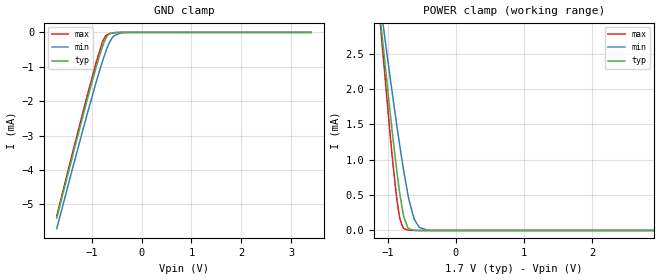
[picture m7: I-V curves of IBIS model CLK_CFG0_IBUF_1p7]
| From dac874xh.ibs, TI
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|   CLK_CFG0_IBUF_1p7 Model
[Model]   CLK_CFG0_IBUF_1p7
Model_type   Input
Vinl = 0.51
Vinh = 1.19
|   typ   min   max
C_comp   1.23168E-13  1.77948E-14  2.05096E-13
| Where nom  PVT is Nominal Process, 1.7V, 27C
|   Fast PVT is Strong Process,  1.701V, -40C
|   Slow PVT is Weak Process,   1.699V, 150C
[Model spec]
|subparameter
Vinl   0.51   0.5097   0.5103
Vinh   1.19   1.1893   1.1907
[Voltage Range]   1.7   1.699   1.701
[Temperature Range]   27   150   -40
[Power Clamp Reference]   1.7   1.699   1.701
[GND Clamp Reference]   0   0   0
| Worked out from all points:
|   GND clamp passes 1 mA (typ) near -0.91 V on its own axis
|   POWER clamp passes 1 mA (typ) near -0.89 V on its own axis
[GND Clamp]
|   Voltage   I(typ)   I(min)   I(max)
-1.7V     -5.395mA   -5.705mA   -5.337mA
-1.348V   -3.396mA   -3.765mA   -3.303mA
-1.088V   -1.954mA   -2.366mA   -1.834mA
-914.6mV  -1.037mA   -1.472mA   -898.7uA
-802.4mV  -500.1uA   -929.6uA   -361.7uA
-741.2mV  -257.3uA   -658.1uA   -150.9uA
-685.1mV  -103.7uA   -436.3uA   -64.17uA
-603.5mV  -20.81uA   -192.8uA   -23.72uA
-532.1mV  -4.928uA   -82.73uA   -6.835uA
-419.9mV  -241.9nA   -22.06uA   -280.1nA
-261.8mV  0A         -801.4nA   0A
3.4V      0A         0A         0A
[POWER Clamp]
|   Voltage   I(typ)   I(min)   I(max)
-1.7V     8.86mA     7.737mA    9.912mA
-1.098V   2.909mA    3.136mA    2.814mA
-965.6mV  1.682mA    2.174mA    1.371mA
-909.5mV  1.194mA    1.781mA    819.5uA
-868.7mV  860.8uA    1.503mA    469.3uA
-817.7mV  489.8uA    1.168mA    154.7uA
-761.6mV  185.6uA    823.9uA    27.94uA
-705.5mV  41.45uA    519.2uA    6.318uA
-608.6mV  1.612uA    154.1uA    483.3nA
-537.2mV  123.9nA    45.24uA    29.46nA
-419.9mV  0A         3.876uA    0A
3.4V      0A         0A         0A
